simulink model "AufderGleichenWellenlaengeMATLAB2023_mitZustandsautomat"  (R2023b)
settings: Solver=FixedStepDiscrete  StartTime=0.0  StopTime=inf  FixedStep=0.1  RelTol=1e-3
libraries: simulink x2, dspstat3 x1, arduinosensorlib x1

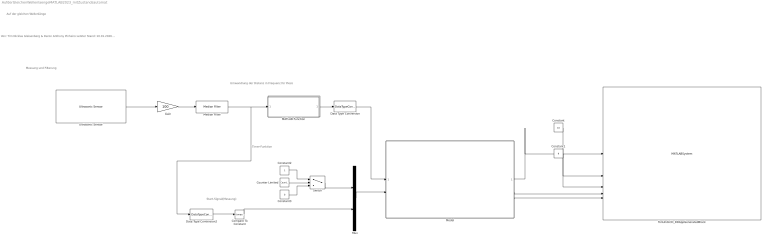
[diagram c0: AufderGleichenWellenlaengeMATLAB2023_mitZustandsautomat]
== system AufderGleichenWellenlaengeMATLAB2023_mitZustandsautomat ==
  note: Von: Tim Nicklas Gleisenberg & Deron Anthony Pinheiro Letzter Stand: 10.01.2026 Benötigte Pakete: Arduino Support Package, Embedded Coder, Signal Processing Toolbox
  note: Auf der gleichen Wellenlänge
  note: Umwandlung der Distanz in Frequenz für Piezo
  note: Messung und Filterung
  note: Start-Signal(Messung)
  note: Timer-Funktion
  Compare To Constant : simulink/Logic and Bit Operations/Compare To Constant  relop=<=  const=50  OutDataTypeStr=uint8
  Constant : Constant  Value=10  OutDataTypeStr=uint8
  Constant1 : Constant  Value=9  OutDataTypeStr=uint8
  Constant2 : Constant
  Constant3 : Constant  Value=0
  Counter Limited : simulink/Sources/Counter Limited  uplimit=2  tsamp=-1
  Data Type Conversion : DataTypeConversion  OutDataTypeStr=uint16
  Data Type Conversion2 : DataTypeConversion  OutDataTypeStr=uint16
  Gain : Gain  Gain=100
  MATLAB Function : MATLAB Function  TreatAsAtomicUnit=on
  Median Filter : dspstat3/Median Filter  WindowLength=10  SimulateUsing=Interpreted execution
  Model : ModelReference  ModelNameDialog=Zustandsautomat.slx  SimulationMode=Normal  ModelReferenceVersion=1.26
  Mux : Mux  Inputs=2
  Switch : Switch  Threshold=1  OutDataTypeStr=uint8
  TonUndLCD_DDAppGeneratedBlock : MATLABSystem  System=TonUndLCD  SampleTime=-1
  Ultrasonic Sensor : arduinosensorlib/Ultrasonic Sensor  NumSignalPins=2  TrigPin=4  EchoPin=5  SignalPin=3  SampleTime_=0.1  blockPlatform=ARDUINO
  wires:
  Ultrasonic Sensor/1 -> Gain/1
  Gain/1 -> Median Filter/1
  Mux/1 -> Model/2
  Constant1/1 -> TonUndLCD_DDAppGeneratedBlock/3
  Constant/1 -> TonUndLCD_DDAppGeneratedBlock/2
  Compare To Constant/1 -> Mux/2
  Counter Limited/1 -> Switch/2
  Switch/1 -> Mux/1
  Data Type Conversion/1 -> Model/1
  Median Filter/1 -> Data Type Conversion2/1, MATLAB Function/1(Distanz)
  MATLAB Function/1(Frequenz) -> Data Type Conversion/1
  Model/1 -> TonUndLCD_DDAppGeneratedBlock/1
  Data Type Conversion2/1 -> Compare To Constant/1
  Constant2/1 -> Switch/1
  Constant3/1 -> Switch/3
  Model/3 -> TonUndLCD_DDAppGeneratedBlock/5
  Model/2 -> TonUndLCD_DDAppGeneratedBlock/4

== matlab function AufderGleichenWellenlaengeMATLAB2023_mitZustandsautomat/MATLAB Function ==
function Frequenz = fcn(Distanz)

if Distanz>50
    Frequenz=0;


elseif Distanz>45
      Frequenz=3000;%65 


elseif Distanz>40 
   Frequenz=3100;  %73


elseif Distanz>35
    Frequenz=3200;%82


elseif Distanz>30
    Frequenz=3300;%87


elseif Distanz>25
    Frequenz=3400;%98


 elseif Distanz>20
    Frequenz=3500;%110


 elseif Distanz>15
    Frequenz=3600;%123


 elseif Distanz>10
    Frequenz=3700;%131


 elseif Distanz>5
    Frequenz=3750;  %196 y 4200 4000 3800 3600 3400 3200 3000 2400 2200 




elseif Distanz<=5
    Frequenz=0;
else Frequenz=0;

end
